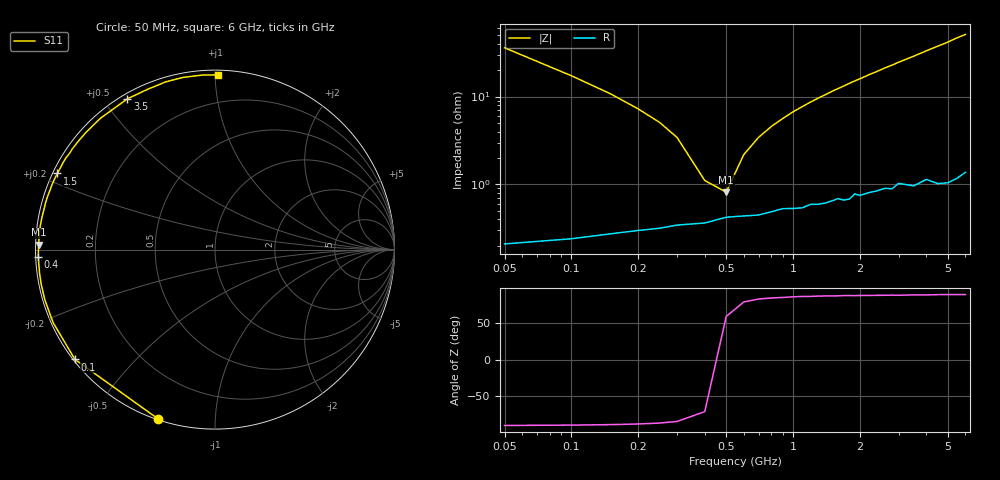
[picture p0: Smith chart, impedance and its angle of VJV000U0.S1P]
! Infineon Technologies  Discrete & RF Semiconductors
! BB 914
! Si Tuning Diode in SOT23
! VR = 0 V
! S-Parameters:  July  1999
# GHz  S  MA  R  50
!  f  S11
! GHz  MAG  ANG
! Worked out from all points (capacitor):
!   34 points, 50 MHz to 6 GHz, reference 50 ohm
!   read as one part to ground: C = 87.8 pF near 50 MHz
!   lowest |Z| = 816 mohm at 500 MHz (marker M1)
!   series resonance near 460 MHz, so ESL is about 1.4 nH
!   S11 on the Smith chart (normalised r, x): 50 MHz: 0.00, -0.72; 100 MHz: 0.00, -0.35; 400 MHz: 0.01, -0.02; 1.5 GHz: 0.01, +0.23; 3.5 GHz: 0.02, +0.57; 6 GHz: 0.03, +1.02
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0.05  0.9945 -108.7
0.1  0.9914 -141.9
0.15  0.9896 -155.7
0.2  0.9883 -163.5
0.25  0.9875 -168.4
0.3  0.9864 -172.2
0.4  0.9856 -177.6
0.5  0.9832 178.4
0.6  0.9827 175.1
0.7  0.9823 172.2
0.8  0.9808 169.6
1.1  0.979 162.6
1.5  0.9756 154.2
1.6  0.9743 152.3
1.7  0.9755 150.4
1.9  0.9718 146.5
2  0.973 144.8
2.2  0.9718 141.0
2.4  0.971 137.7
2.6  0.9698 134.1
2.8  0.9709 131.0
3  0.9674 127.6
3.5  0.9715 120.2
4  0.9688 112.9
4.5  0.9741 106.3
5  0.9756 100.4
5.5  0.9752 94.0
6  0.9734 89.0
